(* Logix 5000 Rung export; software revision 33.00 *)

TYPE Banner_IOL_Device :
STRUCT
   Initial_Global_Read : BOOL;
   Command : SINT;
   Data : Banner_IOL_Device_Index;
   Reset : BOOL;
END_STRUCT
END_TYPE

TYPE Banner_IOL_Device_Index :
STRUCT
   Index : Banner_IOL_Device_SubIndex[32];
END_STRUCT
END_TYPE

TYPE Banner_IOL_Device_SubIndex :
STRUCT
   Sub : DINT[34];
END_STRUCT
END_TYPE

TYPE Banner_IOL_Rules :
STRUCT
   Byte_Pos : SINT;   // Byte Position to read from or write data to.
   Multi : SINT;   // Determines if a multiple byte length index is being accessed. Use 2 for 2 bytes length, 3 for 3 byte length, etc..
   Sub_Index : SINT;
   Signed : SINT;   // 0=unsigned, 1=signed
END_STRUCT
END_TYPE

TYPE Banner_IOL_Rules_Array :
STRUCT
   Length : DINT;
   Settings : Banner_IOL_Rules_SettingsArray[32];
END_STRUCT
END_TYPE

TYPE Banner_IOL_Rules_SettingsArray :
STRUCT
   Index : DINT;
   Num_Op : INT;   // Number of Operations to read/write Index.
   Total_Bytes : INT;
   RW : SINT;   // 0 = Read Only, 1 = Write Only, 2 = Read or Write
   Rules : Banner_IOL_Rules[34];   // Sub Index Position in IODD.
END_STRUCT
END_TYPE

VAR_GLOBAL   (* controller tags *)
   R95C_MDR_Data : Banner_IOL_Device;
        .DATA.INDEX[2]   // Direct Parameters 1
        .DATA.INDEX[2].SUB[1]   // Reserved
        .DATA.INDEX[2].SUB[2]   // Master Cycle Time
        .DATA.INDEX[2].SUB[3]   // Min Cycle Time
        .DATA.INDEX[2].SUB[4]   // M Sequence Capability
        .DATA.INDEX[2].SUB[5]   // IO-Link Version ID
        .DATA.INDEX[2].SUB[6]   // Process Data Input Length
        .DATA.INDEX[2].SUB[7]   // Process Data Output Length
        .DATA.INDEX[2].SUB[8]   // Vendor ID
        .DATA.INDEX[2].SUB[9]   // Device ID
        .DATA.INDEX[3]   // Standard Command
        .DATA.INDEX[3].SUB[1]   // Standard Command: 126=Locator Start, 127=Locator Stop, 129=Application Reset, 164=Reset All Metrics
        .DATA.INDEX[4]   // Serial Number
        .DATA.INDEX[4].SUB[1]   // SN1
        .DATA.INDEX[4].SUB[2]   // SN2
        .DATA.INDEX[4].SUB[3]   // SN3
        .DATA.INDEX[4].SUB[4]   // SN4
        .DATA.INDEX[4].SUB[5]   // SN5
        .DATA.INDEX[4].SUB[6]   // SN6
        .DATA.INDEX[4].SUB[7]   // SN7
        .DATA.INDEX[4].SUB[8]   // SN8
        .DATA.INDEX[4].SUB[9]   // SN9
        .DATA.INDEX[4].SUB[10]   // SN10
        .DATA.INDEX[4].SUB[11]   // SN11
        .DATA.INDEX[4].SUB[12]   // SN12
        .DATA.INDEX[4].SUB[13]   // SN13
        .DATA.INDEX[4].SUB[14]   // SN14
        .DATA.INDEX[4].SUB[15]   // SN15
        .DATA.INDEX[4].SUB[16]   // SN16
        .DATA.INDEX[5]   // All Time Run Time
        .DATA.INDEX[6]   // Resettable Run Time
        .DATA.INDEX[7]   // IO Metrics Port 1
        .DATA.INDEX[7].SUB[1]   // P1 Discrete 1 Count
        .DATA.INDEX[7].SUB[2]   // P1 Discrete 1 Duration
        .DATA.INDEX[7].SUB[3]   // P1 Discrete 1 Events Per Minute
        .DATA.INDEX[7].SUB[4]   // P1 Discrete 1 Totalizer Counter
        .DATA.INDEX[7].SUB[5]   // P1 Discrete 2 Count
        .DATA.INDEX[7].SUB[6]   // P1 Discrete 2 Duration
        .DATA.INDEX[7].SUB[7]   // P1 Discrete 2 Events Per Minute
        .DATA.INDEX[7].SUB[8]   // P! Discrete 2 Totalizer Counter
        .DATA.INDEX[8]   // IO Metrics Port 2
        .DATA.INDEX[8].SUB[1]   // P2 Discrete 1 Count
        .DATA.INDEX[8].SUB[2]   // P2 Discrete 1 Duration
        .DATA.INDEX[8].SUB[3]   // P2 Discrete 1 Events Per Minute
        .DATA.INDEX[8].SUB[4]   // P2 Discrete 1 Totalizer Counter
        .DATA.INDEX[8].SUB[5]   // P2 Discrete 2 Count
        .DATA.INDEX[8].SUB[6]   // P2 Discrete 2 Duration
        .DATA.INDEX[8].SUB[7]   // P2 Discrete 2 Events Per Minute
        .DATA.INDEX[8].SUB[8]   // P2 Discrete 2 Totalizer Counter
        .DATA.INDEX[9]   // IO Metrics Port 3
        .DATA.INDEX[9].SUB[1]   // P3 Discrete 1 Count
        .DATA.INDEX[9].SUB[2]   // P3 Discrete 1 Duration
        .DATA.INDEX[9].SUB[3]   // P3 Discrete 1 Events Per Minute
        .DATA.INDEX[9].SUB[4]   // P3 Discrete 1 Totalizer Counter
        .DATA.INDEX[9].SUB[5]   // P3 Discrete 2 Count
        .DATA.INDEX[9].SUB[6]   // P3 Discrete 2 Duration
        .DATA.INDEX[9].SUB[7]   // P3 Discrete 2 Events Per Minute
        .DATA.INDEX[9].SUB[8]   // P3 Discrete 2 Totalizer Counter
        .DATA.INDEX[10]   // IO Metrics Port 4
        .DATA.INDEX[10].SUB[1]   // P4 Discrete 1 Count
        .DATA.INDEX[10].SUB[2]   // P4 Discrete 1 Duration
        .DATA.INDEX[10].SUB[3]   // P4 Discrete 1 Events Per Minute
        .DATA.INDEX[10].SUB[4]   // P4 Discrete 1 Totalizer Counter
        .DATA.INDEX[10].SUB[5]   // P4 Discrete 2 Count
        .DATA.INDEX[10].SUB[6]   // P4 Discrete 2 Duration
        .DATA.INDEX[10].SUB[7]   // P4 Discrete 2 Events Per Minute
        .DATA.INDEX[10].SUB[8]   // P4 Discrete 2 Totalizer Counter
        .DATA.INDEX[11]   // Input Configuration
        .DATA.INDEX[11].SUB[1]   // Wire Mode: 0=BannerBus, 1=Discrete Input
        .DATA.INDEX[12]   // Motor Run Time Configuration
        .DATA.INDEX[12].SUB[1]   // Motor Current On Setting
        .DATA.INDEX[12].SUB[2]   // Resettable Motor 1 Run Time (value*.25 hrs)
        .DATA.INDEX[12].SUB[3]   // Resettable Motor 2 Run Time (value*.25 hrs)
        .DATA.INDEX[12].SUB[4]   // Resettable Motor 3 Run Time (value*.25 hrs)
        .DATA.INDEX[12].SUB[5]   // Resettable Motor 4 Run Time (value*.25 hrs)
        .DATA.INDEX[13]   // Selectable Metric Reset
        .DATA.INDEX[13].SUB[1]   // Port Discrete Data: 0=Do Not Reset
        .DATA.INDEX[13].SUB[9]   // P1 Discrete 1 Reset Count
        .DATA.INDEX[13].SUB[10]   // P1 Discrete 2 Reset Count
        .DATA.INDEX[13].SUB[11]   // P2 Discrete 1 Reset Count
        .DATA.INDEX[13].SUB[12]   // P2 Discrete 2 Reset Count
        .DATA.INDEX[13].SUB[13]   // P3 Discrete 1 Reset Count
        .DATA.INDEX[13].SUB[14]   // P3 Discrete 2 Reset Count
        .DATA.INDEX[13].SUB[15]   // P4 Discrete 1 Reset Count
        .DATA.INDEX[13].SUB[16]   // P4 Discrete 2 Reset Count
        .DATA.INDEX[14]   // Port 1 Configuration
        .DATA.INDEX[14].SUB[1]   // P1 Discrete 1 IO Selection: 0=NPN input, 1=PNP input, 2=NPN output with Pull Up, 3=PNP Output with Pull Down, 4=NPN Output Push Pull, 5=PNP Output Push Pull
        .DATA.INDEX[14].SUB[2]   // P1 Discrete 1 Delay Mode: 0=Disabled, 1=On Off Delay, 2=On One-Shot, 3=Off One-Shot
        .DATA.INDEX[14].SUB[3]   // P1 Discrete 1 Delay Timer 1: On Delay, One-Shot, Pulse-Stretcher Time, or Totalizer.
        .DATA.INDEX[14].SUB[4]   // P1 Discrete 1 Delay Timer 2: Off Delay or Totalizer.
        .DATA.INDEX[14].SUB[5]   // P1 Discrete 2 IO Selection: 0=NPN input, 1=PNP input, 2=NPN output with Pull Up, 3=PNP Output with Pull Down, 4=NPN Output Push Pull, 5=PNP Output Push Pull
        .DATA.INDEX[14].SUB[6]   // P1 Discrete 2 Delay ModeP1 Discrete 1 Delay Mode: 0=Disabled, 1=On Off Delay, 2=On One-Shot, 3=Off One-Shot
        .DATA.INDEX[14].SUB[7]   // P1 Discrete 1 Delay Timer 1: On Delay, One-Shot, Pulse-Stretcher Time, or Totalizer.
        .DATA.INDEX[14].SUB[8]   // P1 Discrete 1 Delay Timer 2: Off Delay or Totalizer.
        .DATA.INDEX[15]   // Port 2 Configuration
        .DATA.INDEX[15].SUB[1]   // P2 Discrete 1 IO Selection: 0=NPN input, 1=PNP input, 2=NPN output with Pull Up, 3=PNP Output with Pull Down, 4=NPN Output Push Pull, 5=PNP Output Push Pull
        .DATA.INDEX[15].SUB[2]   // P2 Discrete 1 Delay Mode: 0=Disabled, 1=On Off Delay, 2=On One-Shot, 3=Off One-Shot
        .DATA.INDEX[15].SUB[3]   // P1 Discrete 1 Delay Timer 1: On Delay, One-Shot, Pulse-Stretcher Time, or Totalizer.
        .DATA.INDEX[15].SUB[4]   // P2 Discrete 1 Delay Timer 2: Off Delay or Totalizer.
        .DATA.INDEX[15].SUB[5]   // P2 Discrete 2 IO Selection: 0=NPN input, 1=PNP input, 2=NPN output with Pull Up, 3=PNP Output with Pull Down, 4=NPN Output Push Pull, 5=PNP Output Push Pull
        .DATA.INDEX[15].SUB[6]   // P2 Discrete 2 Delay Mode: 0=Disabled, 1=On Off Delay, 2=On One-Shot, 3=Off One-Shot
        .DATA.INDEX[15].SUB[7]   // P1 Discrete 1 Delay Timer 1: On Delay, One-Shot, Pulse-Stretcher Time, or Totalizer.
        .DATA.INDEX[15].SUB[8]   // P2 Discrete 2 Delay Timer 2: Off Delay or Totalizer.
        .DATA.INDEX[16]   // Port 3 Configuration
        .DATA.INDEX[16].SUB[1]   // P3 Discrete 1 IO Selection: 0=NPN input, 1=PNP input, 2=NPN output with Pull Up, 3=PNP Output with Pull Down, 4=NPN Output Push Pull, 5=PNP Output Push Pull
        .DATA.INDEX[16].SUB[2]   // P3 Discrete 1 Delay Mode: 0=Disabled, 1=On Off Delay, 2=On One-Shot, 3=Off One-Shot
        .DATA.INDEX[16].SUB[3]   // P1 Discrete 1 Delay Timer 1: On Delay, One-Shot, Pulse-Stretcher Time, or Totalizer.
        .DATA.INDEX[16].SUB[4]   // P3 Discrete 1 Delay Timer 2: Off Delay or Totalizer.
        .DATA.INDEX[16].SUB[5]   // P3 Discrete 2 IO Selection: 0=NPN input, 1=PNP input, 2=NPN output with Pull Up, 3=PNP Output with Pull Down, 4=NPN Output Push Pull, 5=PNP Output Push Pull
        .DATA.INDEX[16].SUB[6]   // P3 Discrete 2 Delay Mode: 0=Disabled, 1=On Off Delay, 2=On One-Shot, 3=Off One-Shot
        .DATA.INDEX[16].SUB[7]   // P1 Discrete 1 Delay Timer 1: On Delay, One-Shot, Pulse-Stretcher Time, or Totalizer.
        .DATA.INDEX[16].SUB[8]   // P3 Discrete 2 Delay Timer 2: Off Delay or Totalizer.
        .DATA.INDEX[17]   // Port 4 Configuration
        .DATA.INDEX[17].SUB[1]   // P4 Discrete 1 IO Selection: 0=NPN input, 1=PNP input, 2=NPN output with Pull Up, 3=PNP Output with Pull Down, 4=NPN Output Push Pull, 5=PNP Output Push Pull
        .DATA.INDEX[17].SUB[2]   // P4 Discrete 1 Delay Mode: 0=Disabled, 1=On Off Delay, 2=On One-Shot, 3=Off One-Shot
        .DATA.INDEX[17].SUB[3]   // P1 Discrete 1 Delay Timer 1: On Delay, One-Shot, Pulse-Stretcher Time, or Totalizer.
        .DATA.INDEX[17].SUB[4]   // P4 Discrete 1 Delay Timer 2: Off Delay or Totalizer.
        .DATA.INDEX[17].SUB[5]   // P4 Discrete 2 IO Selection: 0=NPN input, 1=PNP input, 2=NPN output with Pull Up, 3=PNP Output with Pull Down, 4=NPN Output Push Pull, 5=PNP Output Push Pull
        .DATA.INDEX[17].SUB[6]   // P4 Discrete 2 Delay Mode: 0=Disabled, 1=On Off Delay, 2=On One-Shot, 3=Off One-Shot
        .DATA.INDEX[17].SUB[7]   // P1 Discrete 1 Delay Timer 1: On Delay, One-Shot, Pulse-Stretcher Time, or Totalizer.
        .DATA.INDEX[17].SUB[8]   // P4 Discrete 2 Delay Timer 2: Off Delay or Totalizer.
        .DATA.INDEX[18]   // Motor 1 Control Config
        .DATA.INDEX[18].SUB[1]   // Motor Power Enable: 0=Disabled, 1=Enabled
        .DATA.INDEX[18].SUB[2]   // Max Analog Setting
        .DATA.INDEX[18].SUB[3]   // Max Current Setting
        .DATA.INDEX[18].SUB[4]   // Current In-Rush Delay Setting
        .DATA.INDEX[18].SUB[5]   // Ramp On Delay
        .DATA.INDEX[18].SUB[6]   // Ramp Off Delay
        .DATA.INDEX[19]   // Motor 2 Control Config
        .DATA.INDEX[19].SUB[1]   // Motor Power Enable: 0=Disabled, 1=Enabled
        .DATA.INDEX[19].SUB[2]   // Max Analog Setting
        .DATA.INDEX[19].SUB[3]   // Max Current Setting
        .DATA.INDEX[19].SUB[4]   // Current In-Rush Delay Setting
        .DATA.INDEX[19].SUB[5]   // Ramp On Delay
        .DATA.INDEX[19].SUB[6]   // Ramp Off Delay
        .DATA.INDEX[20]   // Motor 3 Control Config
        .DATA.INDEX[20].SUB[1]   // Motor Power Enable: 0=Disabled, 1=Enabled
        .DATA.INDEX[20].SUB[2]   // Max Analog Setting
        .DATA.INDEX[20].SUB[3]   // Max Current Setting
        .DATA.INDEX[20].SUB[4]   // Current In-Rush Delay Setting
        .DATA.INDEX[20].SUB[5]   // Ramp On Delay
        .DATA.INDEX[20].SUB[6]   // Ramp Off Delay
        .DATA.INDEX[21]   // Motor 4 Control Config
        .DATA.INDEX[21].SUB[1]   // Motor Power Enable: 0=Disabled, 1=Enabled
        .DATA.INDEX[21].SUB[2]   // Max Analog Setting
        .DATA.INDEX[21].SUB[3]   // Max Current Setting
        .DATA.INDEX[21].SUB[4]   // Current In-Rush Delay Setting
        .DATA.INDEX[21].SUB[5]   // Ramp On Delay
        .DATA.INDEX[21].SUB[6]   // Ramp Off Delay
        .DATA.INDEX[22]   // Block Configuration
        .DATA.INDEX[22].SUB[1]   // Temperature High SP
        .DATA.INDEX[22].SUB[2]   // Temperature Scale: 0=F, 1=C
        .DATA.INDEX[22].SUB[3]   // Undervoltage Alarm SP
        .DATA.INDEX[22].SUB[4]   // Overvoltage Alarm SP
        .DATA.INDEX[22].SUB[5]   // Analog Fix Speed Setting
        .DATA.INDEX[23]   // Monitoring
        .DATA.INDEX[23].SUB[1]   // Temperature F Reading
        .DATA.INDEX[23].SUB[2]   // Temperature C Reading
        .DATA.INDEX[23].SUB[3]   // Block Voltage Reading
        .DATA.INDEX[23].SUB[4]   // Motor 1 Current Reading
        .DATA.INDEX[23].SUB[5]   // Motor 2 Current Reading
        .DATA.INDEX[23].SUB[6]   // Motor 3 Current Reading
        .DATA.INDEX[23].SUB[7]   // Motor 4 Current Reading
   R95C_MDR_Rules : Banner_IOL_Rules_Array;
        .SETTINGS[2]   // Direct Parameters 1
        .SETTINGS[2].RULES[0]   // Reserved
        .SETTINGS[2].RULES[1]   // Master Cycle Time
        .SETTINGS[2].RULES[2]   // Min Cycle Time
        .SETTINGS[2].RULES[3]   // M-Sequence Capability
        .SETTINGS[2].RULES[4]   // IO-Link ID
        .SETTINGS[2].RULES[5]   // Process Data Input Length
        .SETTINGS[2].RULES[6]   // Process Data Output Length
        .SETTINGS[2].RULES[7]   // Vendor ID
        .SETTINGS[2].RULES[8]   // Device ID
        .SETTINGS[3]   // Standard Command
        .SETTINGS[3].RULES[0]   // Standard Command
        .SETTINGS[4]   // Serial Number
        .SETTINGS[4].RULES[0]   // SN1
        .SETTINGS[4].RULES[1]   // SN2
        .SETTINGS[4].RULES[2]   // SN3
        .SETTINGS[4].RULES[3]   // SN4
        .SETTINGS[4].RULES[4]   // SN5
        .SETTINGS[4].RULES[5]   // SN6
        .SETTINGS[4].RULES[6]   // SN7
        .SETTINGS[4].RULES[7]   // SN8
        .SETTINGS[4].RULES[8]   // SN9
        .SETTINGS[4].RULES[9]   // SN10
        .SETTINGS[4].RULES[10]   // SN11
        .SETTINGS[4].RULES[11]   // SN12
        .SETTINGS[4].RULES[12]   // SN13
        .SETTINGS[4].RULES[13]   // SN14
        .SETTINGS[4].RULES[14]   // SN15
        .SETTINGS[4].RULES[15]   // SN16
        .SETTINGS[5]   // All Time Run Time
        .SETTINGS[5].RULES[0]   // All Time Run Time
        .SETTINGS[6]   // Resettable Run Time
        .SETTINGS[6].RULES[0]   // Resettable Run Time
        .SETTINGS[7]   // IO Metrics Port 1
        .SETTINGS[7].RULES[0]   // P1 Discrete 1 Count
        .SETTINGS[7].RULES[1]   // P1 Discrete 1 Duration
        .SETTINGS[7].RULES[2]   // P1 Discrete 1 Events Per Minute
        .SETTINGS[7].RULES[3]   // P1 Discrete 1 Totalizer Counter
        .SETTINGS[7].RULES[4]   // P1 Discrete 2 Count
        .SETTINGS[7].RULES[5]   // P1 Discrete 2 Duration
        .SETTINGS[7].RULES[6]   // P1 Discrete 2 Events Per Minute
        .SETTINGS[7].RULES[7]   // P1 Discrete 2 Totalizer Counter
        .SETTINGS[8]   // IO Metrics Port 2
        .SETTINGS[8].RULES[0]   // P2 Discrete 1 Count
        .SETTINGS[8].RULES[1]   // P2 Discrete 1 Duration
        .SETTINGS[8].RULES[2]   // P2 Discrete Events Per Minute
        .SETTINGS[8].RULES[3]   // P2 Discrete 1 Totalizer Counter
        .SETTINGS[8].RULES[4]   // P2 Discrete 2 Count
        .SETTINGS[8].RULES[5]   // P2 Discrete 2 Duration
        .SETTINGS[8].RULES[6]   // P2 Discrete 2 Events Per Minute
        .SETTINGS[8].RULES[7]   // P2 Discrete 2 Totalizer Counter
        .SETTINGS[9]   // IO Metrics Port 3
        .SETTINGS[9].RULES[0]   // P3 Discrete 1 Count
        .SETTINGS[9].RULES[1]   // P3 Discrete 1 Duration
        .SETTINGS[9].RULES[2]   // P3 Discrete 1 Events Per Minute
        .SETTINGS[9].RULES[3]   // P3 Discrete 1 Totalizer Counter
        .SETTINGS[9].RULES[4]   // P3 Discrete 2 Count
        .SETTINGS[9].RULES[5]   // P3 Discrete 2 Duration
        .SETTINGS[9].RULES[6]   // P3 Discrete 2 Events Per Minute
        .SETTINGS[9].RULES[7]   // P3 Discrete 2 Totalizer Counter
        .SETTINGS[10]   // IO Metrics Port 4
        .SETTINGS[10].RULES[0]   // P4 Discrete 1 Count
        .SETTINGS[10].RULES[1]   // P4 Discrete 1 Duration
        .SETTINGS[10].RULES[2]   // P4 Discrete 1 Events Per Minute
        .SETTINGS[10].RULES[3]   // P4 Discrete 1 Totalizer Counter
        .SETTINGS[10].RULES[4]   // P4 Discrete 2 Count
        .SETTINGS[10].RULES[5]   // P4 Discrete 2 Duration
        .SETTINGS[10].RULES[6]   // P4 Discrete 2 Events Per Minute
        .SETTINGS[10].RULES[7]   // P4 Discrete 2 Totalizer Counter
        .SETTINGS[11]   // Input Configuration
        .SETTINGS[11].RULES[0]   // Wire Mode
        .SETTINGS[12]   // Motor Run Time Configuration
        .SETTINGS[12].RULES[0]   // Motor Current On Setting
        .SETTINGS[12].RULES[1]   // Resettable Motor 1 Run Time
        .SETTINGS[12].RULES[2]   // Resettable Motor 2 Run Time
        .SETTINGS[12].RULES[3]   // Resettable Motor 3 Run Time
        .SETTINGS[12].RULES[4]   // Resettable Motor 4 Run Time
        .SETTINGS[13]   // Selectable Metric Reset
        .SETTINGS[13].RULES[0]   // Port Discrete Status: 0=Do Not Reset, 1=Reset.
        .SETTINGS[13].RULES[1]   // P1 Discrete 1 Reset Count
        .SETTINGS[13].RULES[2]   // P1 Discrete 2 Reset Count
        .SETTINGS[13].RULES[3]   // P2 Discrete 1 Reset Count
        .SETTINGS[13].RULES[4]   // P2 Discrete 2 Reset Count
        .SETTINGS[13].RULES[5]   // P3 Discrete 1 Reset Count
        .SETTINGS[13].RULES[6]   // P3 Discrete 2 Reset Count
        .SETTINGS[13].RULES[7]   // P4 Discrete 1 Reset Count
        .SETTINGS[13].RULES[8]   // P4 Discrete 2 Reset Count
        .SETTINGS[14]   // Port 1 Configuration
        .SETTINGS[14].RULES[0]   // Discrete 1 IO Selection
        .SETTINGS[14].RULES[1]   // Discrete 1 Delay Mode
        .SETTINGS[14].RULES[2]   // Discrete 1 Delay Timer 1
        .SETTINGS[14].RULES[3]   // Discrete 1 Delay Timer 2
        .SETTINGS[14].RULES[4]   // Discrete 2 IO Selection
        .SETTINGS[14].RULES[5]   // Discrete 2 Delay Mode
        .SETTINGS[14].RULES[6]   // Discrete 2 Delay Timer 1
        .SETTINGS[14].RULES[7]   // Discrete 2 Delay Timer 2
        .SETTINGS[15]   // Port 2 Configuration
        .SETTINGS[15].RULES[0]   // Discrete 1 IO Selection
        .SETTINGS[15].RULES[1]   // Discrete 1 Delay Mode
        .SETTINGS[15].RULES[2]   // Discrete 1 Delay Timer 1
        .SETTINGS[15].RULES[3]   // Discrete 1 Delay Timer 2
        .SETTINGS[15].RULES[4]   // Discrete 2 IO Selection
        .SETTINGS[15].RULES[5]   // Discrete 2 Delay Mode
        .SETTINGS[15].RULES[6]   // Discrete 2 Delay Timer 1
        .SETTINGS[15].RULES[7]   // Discrete 2 Delay Timer 2
        .SETTINGS[16]   // Port 3 Configuration
        .SETTINGS[16].RULES[0]   // Discrete 1 IO Selection
        .SETTINGS[16].RULES[1]   // Discrete 1 Delay Mode
        .SETTINGS[16].RULES[2]   // Discrete 1 Delay Timer 1
        .SETTINGS[16].RULES[3]   // Discrete 1 Delay Timer 2
        .SETTINGS[16].RULES[4]   // Discrete 2 IO Selection
        .SETTINGS[16].RULES[5]   // Discrete 2 Delay Mode
        .SETTINGS[16].RULES[6]   // Discrete 2 Delay Timer 1
        .SETTINGS[16].RULES[7]   // Discrete 2 Delay Timer 2
        .SETTINGS[17]   // Port 4 Configuration
        .SETTINGS[17].RULES[0]   // Discrete 1 IO Selection
        .SETTINGS[17].RULES[1]   // Discrete 1 Delay Mode
        .SETTINGS[17].RULES[2]   // Discrete 1 Delay Timer 1
        .SETTINGS[17].RULES[3]   // Discrete 1 Delay Timer 2
        .SETTINGS[17].RULES[4]   // Discrete 2 IO Selection
        .SETTINGS[17].RULES[5]   // Discrete 2 Delay Mode
        .SETTINGS[17].RULES[6]   // Discrete 2 Delay Timer 1
        .SETTINGS[17].RULES[7]   // Discrete 2 Delay Timer 2
        .SETTINGS[18]   // Motor 1 Control Config
        .SETTINGS[18].RULES[0]   // Motor Power Enable
        .SETTINGS[18].RULES[1]   // Max Analog Setting
        .SETTINGS[18].RULES[2]   // Max Current Setting
        .SETTINGS[18].RULES[3]   // Current In-Rush Delay Setting
        .SETTINGS[18].RULES[4]   // Ramp On Delay
        .SETTINGS[18].RULES[5]   // Ramp Off Delay
        .SETTINGS[19]   // Motor 2 Control Config
        .SETTINGS[19].RULES[0]   // Motor Power Enable
        .SETTINGS[19].RULES[1]   // Max Analog Setting
        .SETTINGS[19].RULES[2]   // Max Current Setting
        .SETTINGS[19].RULES[3]   // Current In-Rush Delay Setting
        .SETTINGS[19].RULES[4]   // Ramp On Delay
        .SETTINGS[19].RULES[5]   // Ramp Off Delay
        .SETTINGS[20]   // Motor 3 Control Config
        .SETTINGS[20].RULES[0]   // Motor Power Enable
        .SETTINGS[20].RULES[1]   // Max Analog Setting
        .SETTINGS[20].RULES[2]   // Max Current Setting
        .SETTINGS[20].RULES[3]   // Current In-Rush Delay Setting
        .SETTINGS[20].RULES[4]   // Ramp On Delay
        .SETTINGS[20].RULES[5]   // Ramp Off Delay
        .SETTINGS[21]   // Motor 4 Control Config
        .SETTINGS[21].RULES[0]   // Motor Power Enable
        .SETTINGS[21].RULES[1]   // Max Analog Setting
        .SETTINGS[21].RULES[2]   // Max Current Setting
        .SETTINGS[21].RULES[3]   // Current In-Rush Setting
        .SETTINGS[21].RULES[4]   // Ramp On Delay
        .SETTINGS[21].RULES[5]   // Ramp Off Delay
        .SETTINGS[22]   // Block Configuration
        .SETTINGS[22].RULES[0]   // Temperature High SP
        .SETTINGS[22].RULES[1]   // Temperature Scale
        .SETTINGS[22].RULES[2]   // Undervoltage Alarm SP
        .SETTINGS[22].RULES[3]   // Overvoltage Alarm SP
        .SETTINGS[22].RULES[4]   // Analg Fix Speed Setting
        .SETTINGS[23]   // Monitoring
        .SETTINGS[23].RULES[0]   // Temperatue F Reading
        .SETTINGS[23].RULES[1]   // Temperature C Reading
        .SETTINGS[23].RULES[2]   // Block Voltage Reading
        .SETTINGS[23].RULES[3]   // Motor 1 Current Reading
        .SETTINGS[23].RULES[4]   // Motor 2 Current Reading
        .SETTINGS[23].RULES[5]   // Motor 3 Current Reading
        .SETTINGS[23].RULES[6]   // Motor 4 Current Reading
END_VAR

PROGRAM MainProgram

ROUTINE MainRoutine   (* ladder *)
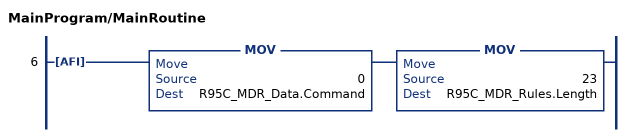
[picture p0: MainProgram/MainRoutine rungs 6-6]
   6: AFI()MOV(0,R95C_MDR_Data.Command)MOV(23,R95C_MDR_Rules.Length);
END_ROUTINE
END_PROGRAM
